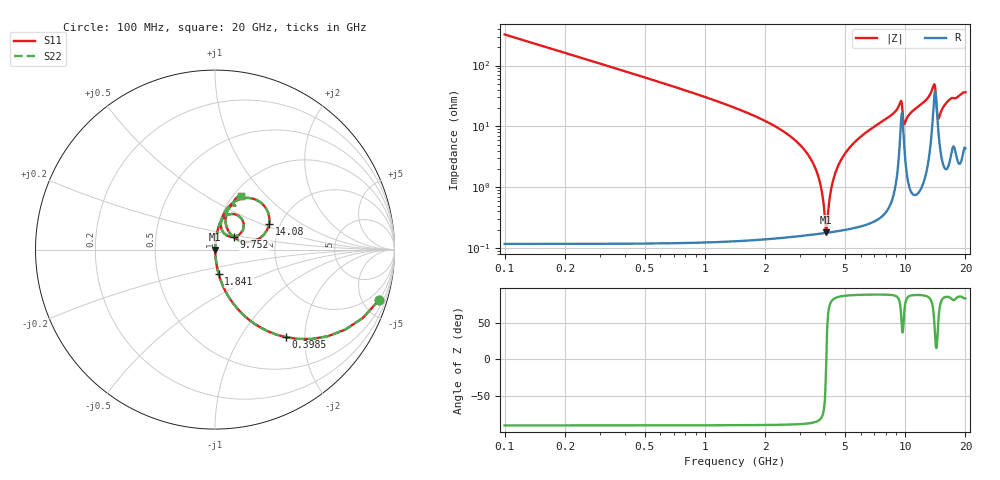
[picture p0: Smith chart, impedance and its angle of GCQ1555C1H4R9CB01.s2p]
!Murata Part Number: GCQ1555C1H4R9CB01
!These Parameters are Measured in Series Mode Connection
!Data Generated on Jan 08, 2026
!  o--ll--o
!Port1  Port2
!  o------o
!Operation Temp=25[degC], DC Bias Voltage=0[V]
!Freq. Start=100[MHz] Stop=20[GHz] 401[Steps]
# Hz S RI R 50
!Freq.(Hz) S11(Real) S11(Imag) S21(Real) S21(Imag) S12(Real) S12(Imag) S22(Real) S22(Imag)
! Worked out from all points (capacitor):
!   401 points, 100 MHz to 20 GHz, reference 50 ohm
!   read as one part in series: C = 4.9 pF near 199.5 MHz
!   lowest |Z| = 182 mohm at 4.03 GHz (marker M1)
!   series resonance near 4.04 GHz, so ESL is about 320 pH
!   S11 on the Smith chart (normalised r, x): 100 MHz: 1.00, -6.49; 398.5 MHz: 1.00, -1.61; 1.841 GHz: 1.00, -0.28; 9.752 GHz: 1.22, +0.18; 14.08 GHz: 1.75, +0.56; 20 GHz: 1.09, +0.72
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1e8  0.9132 -0.2813  0.0868 0.2813  0.0868 0.2813  0.9132 -0.2813
3.985e8  0.3947 -0.488  0.6053 0.488  0.6053 0.488  0.3947 -0.488
8.4625e8  0.1196 -0.3228  0.8804 0.3228  0.8804 0.3228  0.1196 -0.3228
1.84125e9  0.0205 -0.137  0.9795 0.137  0.9795 0.137  0.0205 -0.137
2.83625e9  0.00492 -0.058  0.9951 0.058  0.9951 0.058  0.00492 -0.058
3.43325e9  0.00235 -0.0264  0.9976 0.0264  0.9976 0.0264  0.00235 -0.0264
3.73175e9  0.00188 -0.0129  0.9981 0.0129  0.9981 0.0129  0.00188 -0.0129
4.03025e9  0.00177 -0.000401  0.9982 0.000401  0.9982 0.000401  0.00177 -0.000401
4.12975e9  0.0018 0.00356  0.9982 -0.00356  0.9982 -0.00356  0.0018 0.00356
4.3785e9  0.00201 0.0131  0.998 -0.0131  0.998 -0.0131  0.00201 0.0131
4.7765e9  0.00268 0.0275  0.9973 -0.0275  0.9973 -0.0275  0.00268 0.0275
5.5725e9  0.00504 0.0538  0.995 -0.0538  0.995 -0.0538  0.00504 0.0538
6.7665e9  0.0108 0.0902  0.9892 -0.0902  0.9892 -0.0902  0.0108 0.0902
9.453e9  0.1089 0.1975  0.8911 -0.1975  0.8911 -0.1975  0.1089 0.1975
9.7515e9  0.1062 0.0709  0.8938 -0.0709  0.8938 -0.0709  0.1062 0.0709
1.005e10  0.0375 0.1116  0.9625 -0.1116  0.9625 -0.1116  0.0375 0.1116
1.338325e10  0.1379 0.2813  0.8621 -0.2813  0.8621 -0.2813  0.1379 0.2813
1.378125e10  0.2328 0.2759  0.7672 -0.2759  0.7672 -0.2759  0.2328 0.2759
1.407975e10  0.3014 0.1434  0.6986 -0.1434  0.6986 -0.1434  0.3014 0.1434
1.4627e10  0.0896 0.0829  0.9104 -0.0829  0.9104 -0.0829  0.0896 0.0829
1.67165e10  0.0922 0.2449  0.9078 -0.2449  0.9078 -0.2449  0.0922 0.2449
2e10  0.144 0.2959  0.856 -0.2959  0.856 -0.2959  0.144 0.2959
